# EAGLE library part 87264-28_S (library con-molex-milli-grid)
RECEPTACAL
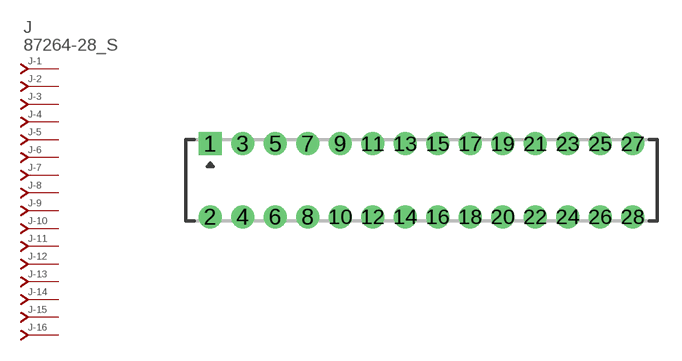
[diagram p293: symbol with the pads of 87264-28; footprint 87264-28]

Designator prefix J; gates -1=J-NV -2=J-N -3=J-N -4=J-N -5=J-N -6=J-N -7=J-N -8=J-N -9=J-N -10=J-N -11=J-N -12=J-N -13=J-N -14=J-N -15=J-N -16=J-N -17=J-N -18=J-N -19=J-N -20=J-N -21=J-N -22=J-N -23=J-N -24=J-N -25=J-N -26=J-N -27=J-N -28=J-N

## 87264-28_S  [87264-28]
1  -1:J  pas
2  -2:J  pas
3  -3:J  pas
4  -4:J  pas
5  -5:J  pas
6  -6:J  pas
7  -7:J  pas
8  -8:J  pas
9  -9:J  pas
10  -10:J  pas
11  -11:J  pas
12  -12:J  pas
13  -13:J  pas
14  -14:J  pas
15  -15:J  pas
16  -16:J  pas
17  -17:J  pas
18  -18:J  pas
19  -19:J  pas
20  -20:J  pas
21  -21:J  pas
22  -22:J  pas
23  -23:J  pas
24  -24:J  pas
25  -25:J  pas
26  -26:J  pas
27  -27:J  pas
28  -28:J  pas

## Footprint 87264-28 (pad centres in mm)
RECEPTACAL Dual Row, Side Entry
drill 0.914 square: 1 -13,2.25
drill 0.914: 2 -13,-2.25; 3 -11,2.25; 4 -11,-2.25; 5 -9,2.25; 6 -9,-2.25; 7 -7,2.25; 8 -7,-2.25; 9 -5,2.25; 10 -5,-2.25; 11 -3,2.25; 12 -3,-2.25; 13 -1,2.25; 14 -1,-2.25; 15 1,2.25; 16 1,-2.25; 17 3,2.25; 18 3,-2.25; 19 5,2.25; 20 5,-2.25; 21 7,2.25; 22 7,-2.25; 23 9,2.25; 24 9,-2.25; 25 11,2.25; 26 11,-2.25; 27 13,2.25; 28 13,-2.25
